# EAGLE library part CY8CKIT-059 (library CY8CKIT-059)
Check availability
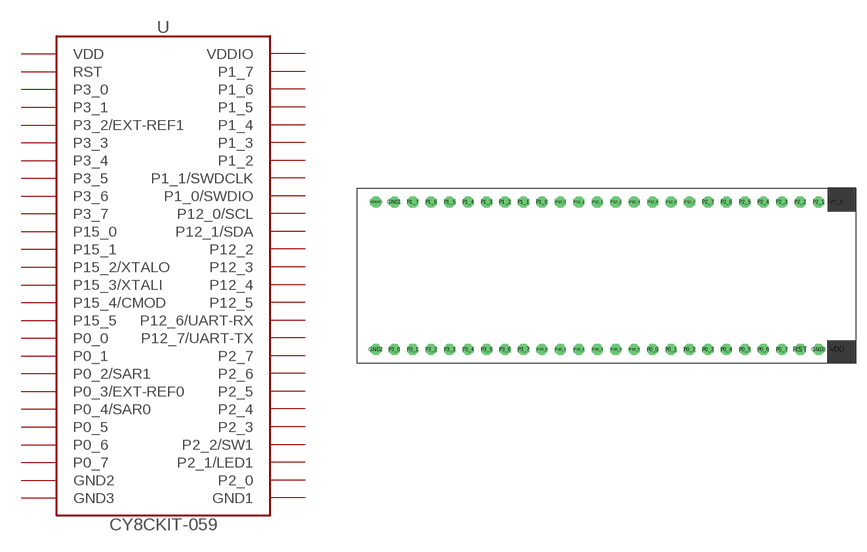
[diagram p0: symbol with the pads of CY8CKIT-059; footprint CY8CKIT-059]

Designator prefix U

## CY8CKIT-059 (Availability: Not in stock; Check_prices: https://www.snapeda.com/parts/CY8CKIT059/Cypress+Semiconductor/view-part/?ref=eda; Description: DEV BOARD, PSOC 5 PROTOTYPING; Silicon Manufacturer:Cypress; No. of Bits:32bit; Silicon Family Name:PSoC 5; Core Architecture:ARM; Core Sub-Architecture:Cortex-M3; Silicon Core Number:CY8C5888LTI; Kit Contents:Dev Board CY8C5888LTI, Quick Start Guide; Product Range:-; SVHC:No SVHC (12-Jan-2017); Features:PSoC 5LP CPU, Snap-away Programmer/Debugger, CapSense, PSoC Creator, 3.3V to 5.5V Supply, Micro-USB; MF: Cypress Semiconductor; MP: CY8CKIT059; Package: None; Price: None; SnapEDA_Link: https://www.snapeda.com/parts/CY8CKIT059/Cypress+Semiconductor/view-part/?ref=snap)  [CY8CKIT-059]
GND1  GND1
GND2  GND2
GND3  GND3
P0_0  P0_0
P0_1  P0_1
P0_2  P0_2/SAR1
P0_3  P0_3/EXT-REF0
P0_4  P0_4/SAR0
P0_5  P0_5
P0_6  P0_6
P0_7  P0_7
P1_0  P1_0/SWDIO
P1_1  P1_1/SWDCLK
P1_2  P1_2
P1_3  P1_3
P1_4  P1_4
P1_5  P1_5
P1_6  P1_6
P1_7  P1_7
P2_0  P2_0
P2_1  P2_1/LED1
P2_2  P2_2/SW1
P2_3  P2_3
P2_4  P2_4
P2_5  P2_5
P2_6  P2_6
P2_7  P2_7
P3_0  P3_0
P3_1  P3_1
P3_2  P3_2/EXT-REF1
P3_3  P3_3
P3_4  P3_4
P3_5  P3_5
P3_6  P3_6
P3_7  P3_7
P12_0  P12_0/SCL
P12_1  P12_1/SDA
P12_2  P12_2
P12_3  P12_3
P12_4  P12_4
P12_5  P12_5
P12_6  P12_6/UART-RX
P12_7  P12_7/UART-TX
P15_0  P15_0
P15_1  P15_1
P15_2  P15_2/XTALO
P15_3  P15_3/XTALI
P15_4  P15_4/CMOD
P15_5  P15_5
RST  RST
VDD  VDD
VDDIO  VDDIO

## Footprint CY8CKIT-059 (pad centres in mm)
drill 1.016 octagon: GND1 -29.21,10.16; GND2 -31.75,-10.16; GND3 29.21,-10.16; P0_0 6.35,-10.16; P0_1 8.89,-10.16; P0_2 11.43,-10.16; P0_3 13.97,-10.16; P0_4 16.51,-10.16; P0_5 19.05,-10.16; P0_6 21.59,-10.16; P0_7 24.13,-10.16; P1_0 -8.89,10.16; P1_1 -11.43,10.16; P1_2 -13.97,10.16; P1_3 -16.51,10.16; P1_4 -19.05,10.16; P1_5 -21.59,10.16; P1_6 -24.13,10.16; P1_7 -26.67,10.16; P2_1 29.21,10.16; P2_2 26.67,10.16; P2_3 24.13,10.16; P2_4 21.59,10.16; P2_5 19.05,10.16; P2_6 16.51,10.16; P2_7 13.97,10.16; P3_0 -29.21,-10.16; P3_1 -26.67,-10.16; P3_2 -24.13,-10.16; P3_3 -21.59,-10.16; P3_4 -19.05,-10.16; P3_5 -16.51,-10.16; P3_6 -13.97,-10.16; P3_7 -11.43,-10.16; P12_0 -6.35,10.16; P12_1 -3.81,10.16; P12_2 -1.27,10.16; P12_3 1.27,10.16; P12_4 3.81,10.16; P12_5 6.35,10.16; P12_6 8.89,10.16; P12_7 11.43,10.16; P15_0 -8.89,-10.16; P15_1 -6.35,-10.16; P15_2 -3.81,-10.16; P15_3 -1.27,-10.16; P15_4 1.27,-10.16; P15_5 3.81,-10.16; RST 26.67,-10.16; VDDIO -31.75,10.16
drill 1.016 square: P2_0 31.75,10.16; VDD 31.75,-10.16

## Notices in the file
This work is licensed under a Creative Commons Attribution-ShareAlike 4.0 International License (CC BY-SA) with Design Exception 1.0
